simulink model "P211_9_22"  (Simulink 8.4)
settings: Solver=ode45  StartTime=0.0  StopTime=10.0  RelTol=1e-3

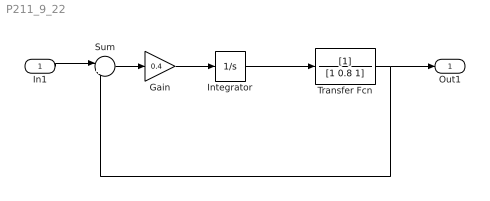
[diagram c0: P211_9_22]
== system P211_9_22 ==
  In1 : Inport
  Gain : Gain  Gain=0.4
  Integrator : Integrator
  Sum : Sum  Inputs=|+-
  Transfer Fcn : TransferFcn  Denominator=[1 0.8 1]
  Out1 : Outport
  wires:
  Transfer Fcn/1 -> Out1/1, Sum/2
  In1/1 -> Sum/1
  Sum/1 -> Gain/1
  Gain/1 -> Integrator/1
  Integrator/1 -> Transfer Fcn/1
